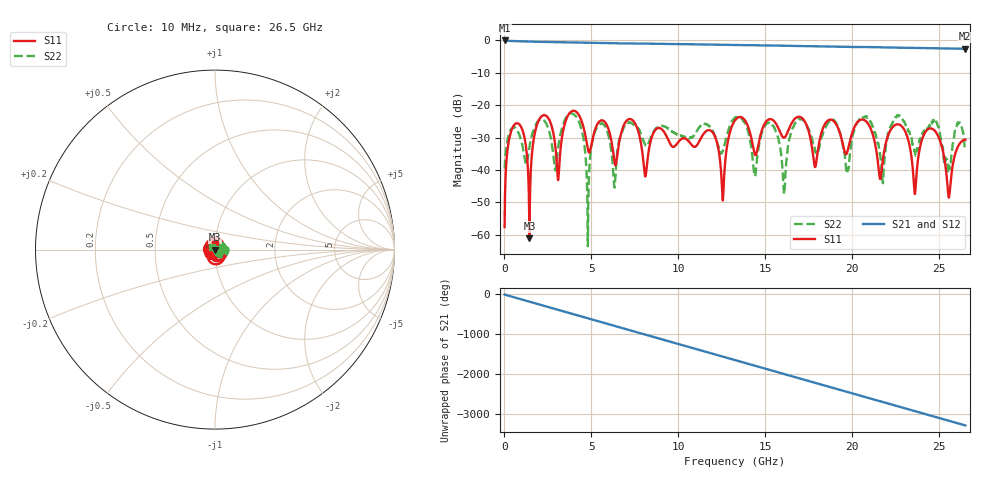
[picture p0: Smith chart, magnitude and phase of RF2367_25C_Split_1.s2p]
!Keysight Technologies,N5245B,MY55451909,A.13.80.08
!Automatic Fixture Removal (AFR)
!Date: Thursday, August 27, 2020, 03:55:56
!S2P File: Measurements: S11,S21,S12,S22:
# MHz S  RI  R 50
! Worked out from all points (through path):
!   2650 points, 10 MHz to 26.5 GHz, reference 50 ohm
!   highest |S21| = -0.01 dB at 10 MHz (marker M1); lowest = -2.6 dB at 26.46 GHz (marker M2)
!   group delay of S21, straight-line fit = 343 ps
!   lowest |S11| = -61.1 dB at 1.44 GHz (marker M3), VSWR 1.00, Z = 50.1 + j0.0112 ohm
!   |S11| at or under -10 dB: start of sweep to end of sweep
!   |S22| runs from -63.5 to -22.5 dB; largest |S21 - S12| = 1.5e-15
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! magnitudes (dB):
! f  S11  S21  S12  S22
! 10 MHz  -57.6  0.0  0.0  -39.5
! 620 MHz  -25.8  -0.2  -0.2  -27.0
! 1.44 GHz  -61.1  -0.3  -0.3  -32.8
! 2.1 GHz  -23.6  -0.4  -0.4  -24.3
! 3.08 GHz  -43.1  -0.5  -0.5  -33.6
! 4.43 GHz  -24.8  -0.7  -0.7  -27.4
! 4.8 GHz  -33.6  -0.7  -0.7  -62.0
! 5.47 GHz  -25.0  -0.8  -0.8  -25.9
! 6.32 GHz  -37.3  -0.9  -0.9  -45.2
! 8.84 GHz  -27.0  -1.0  -1.0  -26.8
! 11.9 GHz  -28.0  -1.3  -1.3  -27.4
! 12.55 GHz  -49.4  -1.3  -1.3  -34.1
! 13.26 GHz  -24.6  -1.4  -1.4  -23.8
! 16.08 GHz  -30.0  -1.6  -1.6  -47.4
! 16.79 GHz  -23.8  -1.7  -1.7  -25.0
! 17.67 GHz  -32.7  -1.8  -1.8  -30.2
! 22.09 GHz  -28.9  -2.2  -2.2  -28.2
! 23.6 GHz  -47.4  -2.3  -2.3  -34.4
! 24.69 GHz  -27.6  -2.4  -2.4  -25.0
! 25.55 GHz  -48.5  -2.5  -2.5  -38.8
! 26.46 GHz  -30.7  -2.6  -2.6  -33.1
! 26.5 GHz  -30.6  -2.5  -2.5  -32.7
